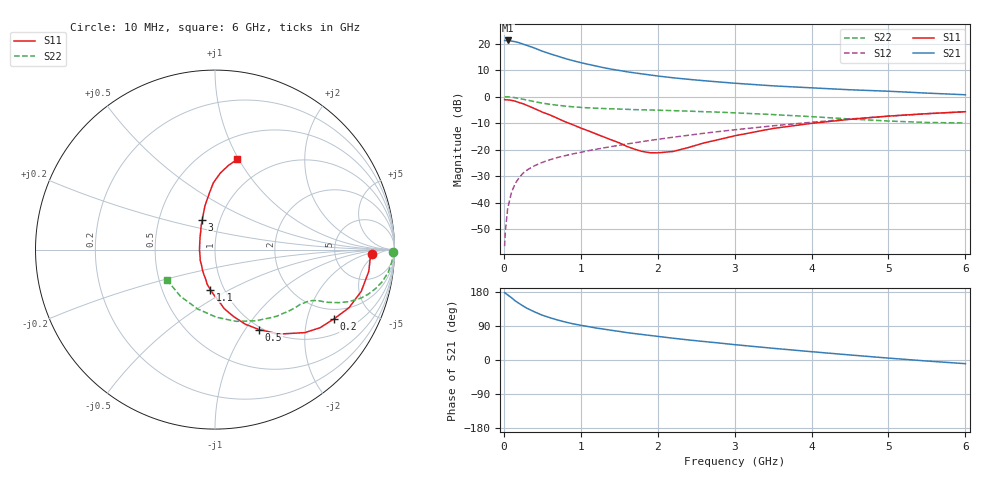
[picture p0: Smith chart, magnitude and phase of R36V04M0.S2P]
! SIEMENS Small Signal Semiconductors
! BFR181
! Si NPN RF Bipolar Junction Transistor in SOT23
! VCE = 6 V  IC = 4 mA
! Common Emitter S-Parameters:  May  1996
# GHz  S  MA  R  50
!  f  S11  S21  S12  S22
! GHz  MAG  ANG  MAG  ANG  MAG  ANG  MAG  ANG
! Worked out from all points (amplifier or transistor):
!   36 points, 10 MHz to 6 GHz, reference 50 ohm
!   highest |S21| = 21.2 dB at 50 MHz (marker M1)
!   |S21| within 3 dB of that: start of sweep to 410.9 MHz
!   unconditionally stable (mu >= 1): 1.268 GHz to 3.12 GHz
!   at 250 MHz: K = 0.36, MSG = 24.3 dB, |S12| = -28.9 dB
!   at 1.4 GHz: K = 1.02, MAG = 13.6 dB, |S12| = -18.9 dB
!   at 6 GHz: K = 0.86, MSG = 3.2 dB, |S12| = -5.7 dB
!   S11 on the Smith chart (normalised r, x): 10 MHz: 14, -3; 200 MHz: 1.57, -2.94; 500 MHz: 0.97, -1.16; 1.1 GHz: 0.86, -0.40; 3 GHz: 0.82, +0.28; 6 GHz: 0.72, +0.98
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0.01  0.8752 -1.7  11.38 178.0  0.0015 101.3  0.9932 -0.7
0.02  0.8661 -3.0  11.32 176.3  0.0029 90.3  0.9869 -1.6
0.05  0.8655 -8.0  11.42 171.8  0.0077 84.4  0.9882 -3.8
0.1  0.8475 -15.9  11.11 164.3  0.0157 83.6  0.9735 -7.5
0.15  0.8142 -23.4  10.8 155.7  0.023 77.1  0.9475 -11.0
0.2  0.7672 -30.2  10.34 149.1  0.0295 73.6  0.9191 -13.8
0.25  0.7296 -36.6  9.743 142.6  0.0358 70.4  0.8881 -16.3
0.3  0.682 -42.7  9.209 136.6  0.0409 68.7  0.8583 -18.3
0.4  0.5909 -52.8  8.207 126.9  0.0495 65.4  0.799 -21.3
0.5  0.5082 -61.2  7.167 118.2  0.0572 63.2  0.75 -23.2
0.6  0.4485 -67.9  6.404 111.6  0.0642 62.0  0.7129 -24.4
0.7  0.3862 -74.6  5.772 105.5  0.0708 61.4  0.6834 -25.4
0.8  0.3325 -81.2  5.2 100.1  0.0767 61.0  0.6588 -25.9
0.9  0.2921 -85.2  4.739 95.5  0.0829 61.2  0.6387 -26.4
1.1  0.2245 -96.8  4.037 88.1  0.095 61.7  0.6111 -27.7
1.6  0.1142 -131.2  2.928 72.3  0.1272 62.1  0.5734 -31.6
2.2  0.0918 158.0  2.256 57.5  0.1707 61.3  0.5411 -38.3
3  0.1813 113.0  1.782 40.5  0.2355 57.3  0.4924 -50.2
3.5  0.2497 103.0  1.589 30.9  0.2799 53.6  0.4561 -60.5
4.5  0.3714 91.5  1.34 13.3  0.3764 44.0  0.3768 -88.9
5.5  0.4743 81.0  1.159 -2.7  0.473 31.7  0.3236 -126.6
6  0.5171 76.2  1.079 -9.7  0.5174 24.8  0.3165 -147.6
